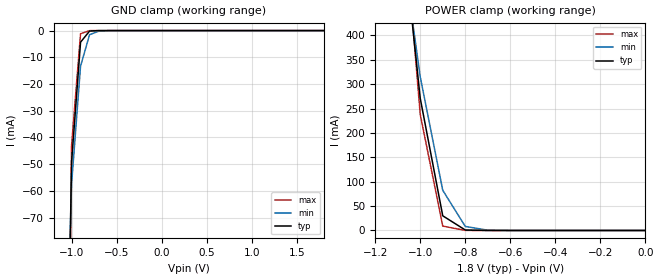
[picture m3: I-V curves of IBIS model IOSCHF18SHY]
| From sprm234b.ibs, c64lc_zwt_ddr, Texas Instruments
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|   Model Cell IOSCHF18SHY
[Model]   IOSCHF18SHY
Model_type   Input
Polarity   Non-Inverting
| signals   A, Y
Vinl = 0.8V
Vinh = 2.0V
|   typ   min   max
C_comp   0.435p   0.374p   0.5435p
|   typ   min   max
[Temperature Range]   25   -40   125
|   typ   min   max
[Voltage Range]   1.80V   1.70V   1.90V
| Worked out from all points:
|   GND clamp passes 1 mA (typ) near -0.82 V on its own axis
|   POWER clamp passes 1 mA (typ) near -0.80 V on its own axis
[GND_clamp]
|   Voltage   I(typ)   I(min)   I(max)
-1.8V     -8.116A    -5.267A    -11.71A
-1.1V     -250.9mA   -179mA     -385.7mA
-1V       -49.35mA   -57.54mA   -43.16mA
-900mV    -4.337mA   -13.31mA   -1.18mA
-800mV    -185.2uA   -1.544mA   -22.65uA
-700mV    -4.758uA   -248uA     -450.2nA
-500mV    -2.448nA   -2.381uA   -643.9pA
1.8V      111pA      22.2pA     133.2pA
[POWER_clamp]
|   Voltage   I(typ)   I(min)   I(max)
-1.8V     4.55A      3.516A     5.705A
-1.1V     710mA      648.6mA    795.8mA
-1V       271.1mA    315.4mA    238mA
-900mV    30.09mA    82.46mA    9.007mA
-800mV    988.1uA    8.286mA    99.36uA
-700mV    26.44uA    606.1uA    857.4nA
0V        1pA        1pA        1pA
